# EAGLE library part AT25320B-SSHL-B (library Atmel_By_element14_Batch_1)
SPI Serial EEPROM
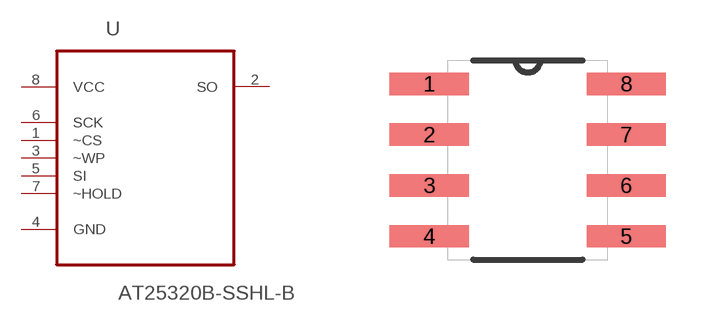
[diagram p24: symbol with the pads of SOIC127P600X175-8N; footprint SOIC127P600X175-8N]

Designator prefix U

## AT25320B-SSHL-B (MPN: AT25320B-SSHL-B; OC_FARNELL: 1841578; OC_NEWARK: 12T1359; PACKAGE: SOIC-8; SUPPLIER: Atmel)  [SOIC127P600X175-8N]
1  ~CS  in
2  SO  out
3  ~WP  in
4  GND  pas
5  SI  in
6  SCK  in
7  ~HOLD  in
8  VCC  pwr

## Footprint SOIC127P600X175-8N (pad centres in mm)
smd 1.981 x 0.559: 1 -2.464,1.905; 2 -2.464,0.635; 3 -2.464,-0.635; 4 -2.464,-1.905; 5 2.464,-1.905; 6 2.464,-0.635; 7 2.464,0.635; 8 2.464,1.905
